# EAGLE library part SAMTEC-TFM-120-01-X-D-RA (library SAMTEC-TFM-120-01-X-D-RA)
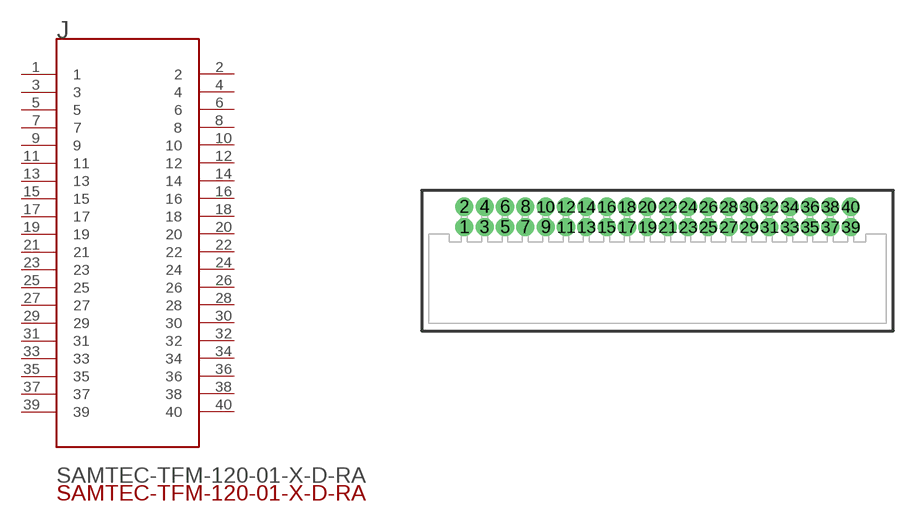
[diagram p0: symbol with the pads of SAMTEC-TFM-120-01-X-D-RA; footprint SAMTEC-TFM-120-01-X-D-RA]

Designator prefix J

## SAMTEC-TFM-120-01-X-D-RA  [SAMTEC-TFM-120-01-X-D-RA]
1  1  pas
2  2  pas
3  3  pas
4  4  pas
5  5  pas
6  6  pas
7  7  pas
8  8  pas
9  9  pas
10  10  pas
11  11  pas
12  12  pas
13  13  pas
14  14  pas
15  15  pas
16  16  pas
17  17  pas
18  18  pas
19  19  pas
20  20  pas
21  21  pas
22  22  pas
23  23  pas
24  24  pas
25  25  pas
26  26  pas
27  27  pas
28  28  pas
29  29  pas
30  30  pas
31  31  pas
32  32  pas
33  33  pas
34  34  pas
35  35  pas
36  36  pas
37  37  pas
38  38  pas
39  39  pas
40  40  pas

## Footprint SAMTEC-TFM-120-01-X-D-RA (pad centres in mm)
translated Allegro footprint
drill 0.635 pad 1.016: 1 -12.065,3.238; 2 -12.065,4.508; 3 -10.795,3.238; 4 -10.795,4.508; 5 -9.525,3.238; 6 -9.525,4.508; 7 -8.255,3.238; 8 -8.255,4.508; 9 -6.985,3.238; 10 -6.985,4.508; 11 -5.715,3.238; 12 -5.715,4.508; 13 -4.445,3.238; 14 -4.445,4.508; 15 -3.175,3.238; 16 -3.175,4.508; 17 -1.905,3.238; 18 -1.905,4.508; 19 -0.635,3.238; 20 -0.635,4.508; 21 0.635,3.238; 22 0.635,4.508; 23 1.905,3.238; 24 1.905,4.508; 25 3.175,3.238; 26 3.175,4.508; 27 4.445,3.238; 28 4.445,4.508; 29 5.715,3.238; 30 5.715,4.508; 31 6.985,3.238; 32 6.985,4.508; 33 8.255,3.238; 34 8.255,4.508; 35 9.525,3.238; 36 9.525,4.508; 37 10.795,3.238; 38 10.795,4.508; 39 12.065,3.238; 40 12.065,4.508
